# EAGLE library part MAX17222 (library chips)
Very high efficiency, very low power boost converter suitable for EH applications
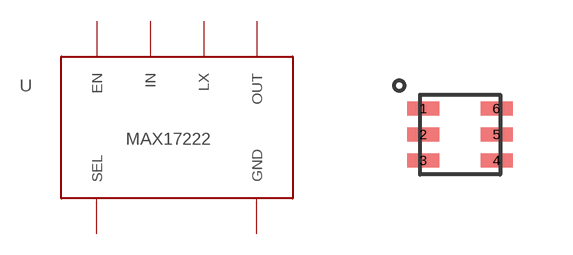
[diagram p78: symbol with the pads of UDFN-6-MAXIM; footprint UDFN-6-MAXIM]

Designator prefix U

## MAX17222 (DIGIKEY: MAX17222ELT+TCT-ND; MANUFACTURER: MAXIM INTEGRATED; MPN: MAX17222ELT+T)  [UDFN-6-MAXIM]
1  OUT
2  LX
3  GND
4  SEL
5  IN
6  EN

## Footprint UDFN-6-MAXIM (pad centres in mm)
smd 0.8 x 0.35: 1 -0.915,0.65; 2 -0.915,0; 3 -0.915,-0.65; 4 0.915,-0.65; 5 0.915,0; 6 0.915,0.65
